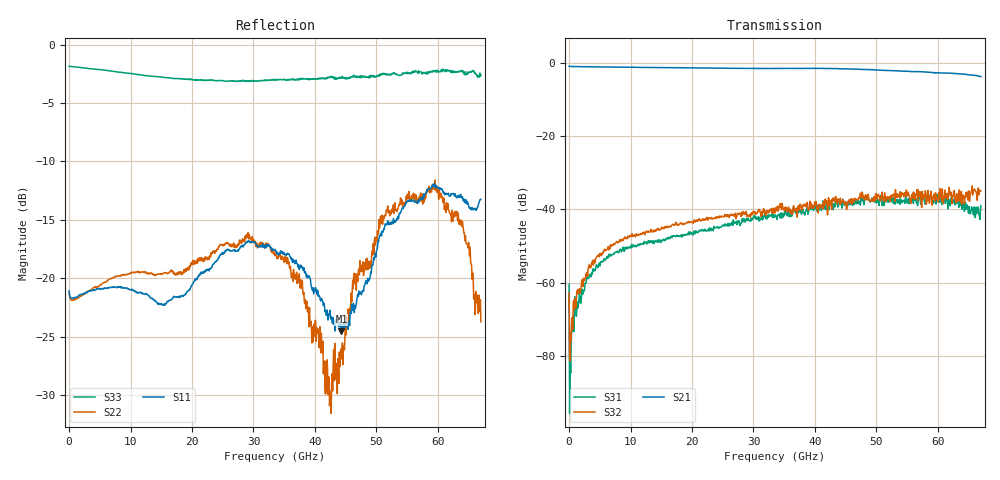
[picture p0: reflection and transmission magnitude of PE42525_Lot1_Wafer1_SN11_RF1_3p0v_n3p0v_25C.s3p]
!Keysight Technologies,N5227A,US51270237,A.10.43.00
!Date: Friday, September 16, 2016 08:58:40
!Correction: S11(Full 3 Port(1,2,3))
!S12(Full 3 Port(1,2,3))
!S13(Full 3 Port(1,2,3))
!S21(Full 3 Port(1,2,3))
!S22(Full 3 Port(1,2,3))
!S23(Full 3 Port(1,2,3))
!S31(Full 3 Port(1,2,3))
!S32(Full 3 Port(1,2,3))
!S33(Full 3 Port(1,2,3))
!S3P File: Measurements: <S11,S12,S13>,
!<S21,S22,S23>,
!<S31,S32,S33>:
# Hz S  dB  R 50
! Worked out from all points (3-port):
!   801 points, 10 MHz to 67 GHz, reference 50 ohm
!   strongest paths, dB at 10 MHz, 16.76 GHz, 33.51 GHz, 50.25 GHz, 67 GHz:
!     S21: -0.8, -1.2, -1.5, -1.9, -3.7
!     S32: -62.9, -44.2, -41.0, -36.4, -35.0
!     S31: -60.4, -47.7, -41.6, -37.3, -38.9
!   lowest |S11| = -24.5 dB at 44.31 GHz (marker M1), VSWR 1.13, Z = 47.2 - j5.07 ohm
!   |S11| at or under -10 dB: start of sweep to end of sweep
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1e7  -21.09 -0.6  -0.81 -0.2  -56.48 79.5
     -0.83 -0.1  -21.20 -0.4  -59.97 -54.5
     -60.43 49.4  -62.89 138.5  -1.84 179.8
4.286875e8  -21.70 -5.5  -0.92 -4.7  -71.86 93.8
            -0.92 -4.6  -21.90 -5.7  -69.49 62.2
            -71.16 87.8  -71.32 103.4  -1.87 176.4
8.802438e9  -20.80 -97.3  -1.11 -89.4  -50.51 3.1
            -1.11 -89.4  -19.70 -94.1  -47.87 -3.3
            -50.34 2.6  -48.46 -2.8  -2.41 110.3
1.759488e10  -21.66 -144.6  -1.25 -178.1  -47.34 -71.9
             -1.26 -178.1  -19.71 -146.8  -44.42 -86.0
             -47.39 -71.2  -44.31 -85.3  -2.90 39.1
2.588489e10  -17.52 161.5  -1.40 97.8  -43.98 -145.4
             -1.40 97.8  -16.98 171.2  -41.52 -161.7
             -43.83 -144.9  -41.46 -161.8  -3.12 -31.8
3.3505e10  -17.54 75.0  -1.47 20.0  -42.41 134.2
           -1.47 19.9  -18.07 100.5  -40.29 138.8
           -41.56 137.5  -40.96 134.6  -2.99 -96.9
4.430714e10  -24.55 -115.6  -1.54 -95.0  -37.71 39.4
             -1.55 -95.1  -26.92 -127.9  -38.47 22.5
             -38.43 38.1  -38.19 30.5  -2.87 174.3
5.134109e10  -15.61 90.0  -1.98 -172.2  -38.12 -33.3
             -1.97 -172.4  -14.64 122.7  -35.56 -38.5
             -38.21 -28.7  -35.44 -38.4  -2.49 121.0
5.837504e10  -12.36 12.3  -2.45 108.8  -37.20 -92.2
             -2.51 108.5  -12.36 44.3  -36.42 -97.1
             -37.48 -93.8  -34.81 -108.5  -2.52 70.4
6.7e10  -13.24 -31.4  -3.65 1.8  -40.16 -160.7
        -3.70 1.5  -23.74 48.6  -36.25 -173.2
        -38.94 -161.9  -34.95 -166.7  -2.62 11.7
